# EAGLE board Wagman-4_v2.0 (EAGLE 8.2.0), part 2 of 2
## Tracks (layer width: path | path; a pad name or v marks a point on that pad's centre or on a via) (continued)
INA3  (via drill 0.3 pad 0.61) (continued)
  Bottom 0.254: SWS001.5 6.7,84.12 R103.1
JTAG_RESET
  Top 0.406: RN1.4 29.06,98.05 R41.1 29.14,96.2 JTAG.10
JTAG_TCK  (via drill 0.3 pad 0.61)
  Top 0.2: U1.28 49.49,72.84 v50.25,73.59
  Top 0.254: JTAG.4 25.07,96.5 26.06,97.5 RN1.2
  Bottom 0.2: JTAG.4 25.07,96.5 26.84,98.28 45.84,98.28 49.88,94.24 49.88,75.59 50.49,74.98 50.49,73.83 v50.25,73.59
JTAG_TDI  (via drill 0.3 pad 0.61)
  Top 0.2: U1.29 47.17,73.34
  Top 0.203: 47.17,73.34 46.87,73.34 v46.76,73.45
  Top 0.254: JTAG.8 27.61,96.61 26.86,97.36 RN1.3
  Bottom 0.2: JTAG.8 27.61,97.05 27.94,97.38 45.34,97.38 48.94,93.78 48.94,74.78 47.78,73.61
  Bottom 0.203: 47.78,73.61 47.61,73.45 v46.76,73.45
JTAG_TDO  (via drill 0.3 pad 0.61)
  Top 0.2: U1.30 49.33,73.84 49.71,74.22 v49.76,74.5
  Bottom 0.2: JTAG.6 26.34,96.88 27.24,97.78 45.64,97.78 49.37,94.05 49.37,74.93 v49.76,74.5
JTAG_TMS  (via drill 0.3 pad 0.61)
  Top 0.2: U1.31 47.11,74.34
  Top 0.203: 47.11,74.34 46.24,74.34 v46.11,74.2
  Top 0.254: JTAG.2 23.79,96.58 RN1.1
  Bottom 0.2: 34.3,96.68 45.24,96.68 48.44,93.48 48.44,75.48 47.65,74.69 | 22.14,95.48 22.59,95.93 JTAG.2
  Bottom 0.203: 34.3,96.68 30.84,96.68 30.27,96.11 30.27,94.48 29.15,93.37 22.45,93.37 22.14,93.67 22.14,95.48 | 47.65,74.69 47.17,74.2 v46.11,74.2
LED0  (via drill 0.3 pad 0.61)
  Top 0.2: U1.68 30.86,75.66 v34.59,71.93
  Top 0.254: R14.1 129.71,88.2 124.23,82.72 107.49,82.72 105.79,82.72 v102.43,79.37
  Bottom 0.2: 62.68,74.87 59.33,71.52 45,71.52 43.48,73.05 35.71,73.05 v34.59,71.93
  Bottom 0.203: v102.43,79.37 101.75,78.68 91.64,78.68 90.57,77.62 71.22,77.62 68.47,74.87 62.68,74.87
LED1  (via drill 0.3 pad 0.61)
  Top 0.254: U1.144 46.36,56.56 v46.84,56.08 | R88.1 113.38,85.06 v113.33,85.01
  Bottom 0.254: v113.33,85.01 107.59,79.27 107.59,69.29 100.48,62.17 91.13,62.17 85.52,56.56 47.31,56.56 v46.84,56.08
LED2  (via drill 0.3 pad 0.61)
  Top 0.254: U1.139 43.86,56.46 44.94,55.38 v46.04,55.38 | R15.1 115.54,85.95 v114.47,84.88
  Bottom 0.254: v46.04,55.38 46.34,55.08 47.84,55.08 48.81,56.05 86.01,56.05 91.53,61.57 100.78,61.57 108.3,69.08 108.3,78.71 v114.47,84.88
LED3  (via drill 0.3 pad 0.61)
  Top 0.254: U1.136 42.36,56.36 43.54,55.18 v44.04,55.18 | R89.1 117.57,86.71 v115.62,84.75
  Bottom 0.254: v44.04,55.18 44.84,55.18 45.57,54.45 48.36,54.45 49.45,55.55 86.51,55.55 91.92,60.96 101.09,60.96 109.01,68.88 109.01,78.15 v115.62,84.75
LED4  (via drill 0.3 pad 0.61)
  Top 0.254: U1.135 41.86,55.96 43.64,54.18 v44.44,54.18 | R37.1 119.61,87.22 v117.14,84.75
  Bottom 0.254: v44.44,54.18 44.94,53.68 48.47,53.68 49.7,54.91 86.87,54.91 92.31,60.35 101.39,60.35 109.72,68.68 109.72,77.62 116.86,84.75 v117.14,84.75
LED5  (via drill 0.3 pad 0.61)
  Top 0.254: U1.134 41.36,55.56 v43.54,53.38 | R90.1 121.51,87.73 v118.54,84.75
  Bottom 0.254: v43.54,53.38 43.84,53.08 48.76,53.08 50.08,54.4 87.46,54.4 92.8,59.74 101.7,59.74 110.33,68.37 110.33,77.27 116.93,83.87 117.65,83.87 v118.54,84.75
LED6  (via drill 0.3 pad 0.61)
  Top 0.254: U1.133 40.86,54.96 v42.34,53.48 | R91.1 123.4,87.97 v120.06,84.63
  Bottom 0.254: v42.34,53.48 43.34,52.48 49.18,52.48 50.59,53.89 87.85,53.89 93.09,59.13 102,59.13 110.94,68.07 110.94,76.91 117.14,83.1 118.54,83.1 v120.06,84.63
LED7  (via drill 0.3 pad 0.61)
  Top 0.254: U1.132 40.36,54.26 v42.24,52.38 | R92.1 125.45,88.62 v121.46,84.63
  Bottom 0.254: v42.24,52.38 42.84,51.78 49.49,51.78 51.1,53.39 88.45,53.39 93.58,58.52 102.31,58.52 111.55,67.76 111.55,76.49 117.53,82.47 119.3,82.47 v121.46,84.63
LED8  (via drill 0.3 pad 0.61)
  Top 0.2: U1.20 56.14,68.84 64.94,77.64 67.74,77.64 v67.99,77.39
  Top 0.254: R93.1 111.22,89.63 v102.05,80.46
  Bottom 0.203: v102.05,80.46 100.73,79.14 91.13,79.14 90.22,78.23 70.71,78.23 69.87,77.39 v67.99,77.39
LED9  (via drill 0.3 pad 0.61)
  Top 0.2: U1.21 55.87,69.34 64.69,78.15 v68.75,78.15
  Top 0.254: R94.1 108.94,88.74 v102,81.81
  Bottom 0.2: 101.53,81.34 v102,81.81
  Bottom 0.203: v68.75,78.15 69.44,78.84 89.91,78.84 90.83,79.75 99.94,79.75 101.53,81.34
LOPS  (via drill 0.3 pad 0.61)
  Top 0.254: v105.84,39.54 105.84,30.53 99.87,24.56 92.81,24.56 90.72,22.47 v90.72,21 | v69.29,10.21 69.14,10.05 R97.2 | U17.11 116.59,68.16 v116.58,68.14 | v105.05,43.89 105.46,44.29 v105.46,46.12
  Top 0.406: JP3.2 67.97,9.9 R97.2
  Bottom 0.254: v90.72,21 90.72,12.11 88.82,10.21 v69.29,10.21 | v116.58,68.14 116.56,68.12 114.55,68.12 103.37,56.94 103.37,48.2 v105.46,46.12 | v105.05,43.89 105.84,43.1 v105.84,39.54
MASTER-RESET  (via drill 0.3 pad 0.61)
  Top 0.2: U1.47 41.36,84.03 43.58,86.25 v43.58,87.17 | v45.92,93.87 45.92,87.57 v46.33,87.17
  Top 0.254: J11.5 v7.34,86.5 36.51,86.5 36.98,86.96 36.98,90.11 37.99,91.13 41.35,91.13 v43.99,93.77 43.64,94.12 43.64,98.48 C41.2 43.99,98.55 | v82.68,81.58 82.74,81.58 83.71,80.61 83.71,78.13 83.98,77.86 U24.1 84.73,77.21 v85.44,76.5 | v136.95,84.22 136.44,84.22 v135.22,83 | v106.88,78.23 v105.25,78.23 | v51.3,86.05 50.59,86.76 46.73,86.76 v46.33,87.17
  Top 0.406: C41.2 RST.2 | R41.2 31.67,98.69 RST.1
  Top 0.61: RST.1 RST.2
  Bottom 0.254: v43.58,87.17 v46.33,87.17 | v51.3,86.05 52.32,85.03 69.39,85.03 72.84,81.58 v82.68,81.58 | v45.92,93.87 45.82,93.77 v43.99,93.77 | U39.4 138.37,85.64 v136.95,84.22 | v135.22,83 125.98,83 122.93,86.05 112.77,86.05 106.88,80.16 v106.88,78.23 | v85.44,76.5 93.77,76.5 95.09,77.82 101.8,77.82 102.51,78.53 104.95,78.53 v105.25,78.23
MFP
  Top 0.406: U2.7 98.83,80.29 R20.1
MR1
  Top 0.254: R4.1 98.09,69.33 Q8.3 98.17,68.64 100.35,66.47 SWS003.1
MR1_3V  (via drill 0.3 pad 0.61)
  Top 0.203: U1.32 46.97,74.84 v46.73,75.08
  Top 0.254: v95.09,81.68 96.01,80.77 96.01,74.16 96.31,73.86 v96.31,72.64 | R3.1 98.36,65.29 Q8.2 98.24,66.55 97.23,67.56 96.52,67.56 96.21,67.86 v96.21,68.88 | v52.22,86.56 51.3,87.47 v47.75,87.47
  Bottom 0.203: v47.75,87.47 47.98,87.24 47.98,76.33 v46.73,75.08
  Bottom 0.254: v96.31,72.64 96.31,68.98 v96.21,68.88 | v52.22,86.56 53.13,85.64 69.9,85.64 73.05,82.49 83.19,82.49 84,81.68 v95.09,81.68
MR2
  Top 0.3: Q1.3 103.67,69.38 103.17,68.88 103.17,65.96 102.66,65.45 101.9,65.45 101.57,65.78 SWS003.2
  Top 0.5: R96.1 105.12,70.26 Q1.3
MR2_3V  (via drill 0.3 pad 0.61)
  Top 0.2: U1.22 55.61,69.84 64.94,79.17 69.13,79.17 | 77.24,76.88 80.82,73.3 v81.94,73.3
  Top 0.203: 69.13,79.17 71.29,77.01 77.11,77.01 77.24,76.88
  Top 0.254: R95.1 106.07,65.95 Q1.2 106.09,67.28 106.09,73.07 105.71,73.45 v97.96,73.45
  Bottom 0.2: v97.96,73.45 82.19,73.45 v81.94,73.3
N$1
  Top 0.254: ON.A 134.03,95.02 133.6,94.58 133.6,92.65 133.97,92.29 RN3.4
N$2
  Bottom 0.254: U37.3 83.76,90.77 83.31,91.23 83.31,92.96 83,93.26 R102.2
N$3
  Top 0.406: L.A R15.2
N$4
  Top 0.406: TX1.A R14.2
N$5
  Top 0.2: U1.51 39.36,79.9 39.86,80.4 39.86,83.88 39.22,84.51 R5.1
N$6
  Top 0.406: R33.2 76.52,64.06 76.74,64.28 77.77,64.28 U18.1
N$7
  Top 0.254: R10.2 37.31,80.94 38.36,79.89 U1.53
N$8
  Top 0.406: U6.4 104.45,19.26 R64.2
N$9
  Top 1.93: F1.1 L6.2
N$10
  Top 0.406: ON1.A R2.2
N$11
  Top 0.2: R6.1 50.58,78.12 49.84,77.38 47.66,77.38 46.78,76.5 44.6,76.5 44.19,76.91 44.19,77.62 43.99,77.82 43.58,77.82 43.36,78.04 U1.43
N$12  (via drill 0.3 pad 0.61)
  Top 0.2: R7.1 47.49,80.43 | U1.42 43.86,80.6 v44.35,81.09
  Top 0.203: 47.49,80.43 46.98,80.43 v46.93,80.48
  Bottom 0.2: v46.93,80.48 44.96,80.48 v44.35,81.09
N$13
  Top 0.5: U25.10 67.57,86.02 R28.1
N$14
  Top 0.254: U20.13 83.42,65.64 83.74,65.32 83.74,62.3 R18.1
N$15
  Top 0.406: U2.2 98.83,91.05 Y3.P$4 97.4,92.04 C15.1
N$16
  Top 0.61: JP9.2 27.29,88.64 U36.3
N$17
  Top 0.406: U2.1 100.1,91.1 Y3.P$1 101.5,92.04 C14.1
N$18
  Top 0.254: U26.3 90.64,71.09 R25.1
N$19  (via drill 0.3 pad 0.61)
  Top 0.254: U21.10 71.23,39.39 v71.24,39.38
  Bottom 0.254: R60.2 71.11,39.25 v71.24,39.38
N$20
  Top 0.203: U20.10 84.49,69.45 85.54,70.51 85.54,72.33 84.15,73.73 R19.1
N$21
  Top 0.813: R21.2 104.83,91.06 D3.K
N$22
  Top 0.406: L7.A R88.2
N$23
  Top 0.61: JP9.1 27.29,91.18 U36.4
N$24
  Top 0.406: U20.4 89.93,68.18 R23.2
N$25
  Top 0.406: L4.A R37.2
N$28
  Top 0.254: U18.4 76.69,68.06 76.37,68.37 76.37,73.33 R34.2
N$29  (via drill 0.3 pad 0.61)
  Top 0.2: v53.89,37.64 53.89,38.76 R38.1
  Top 0.254: J5.1 108.99,13.16 111.93,16.1 v111.93,20.49 | v70.66,24.3 70.15,24.81 70.15,30.32 73.76,33.93 v73.76,36.47
  Bottom 0.254: v111.93,20.49 108.12,24.3 v70.66,24.3 | v53.89,37.64 54.64,37.64 55.81,36.47 v73.76,36.47
N$30
  Top 0.2: U18.10 71.48,69.33 71.22,69.59 71.22,73.76 R35.1
N$31  (via drill 0.3 pad 0.61)
  Top 0.2: v103.93,10.08 103.93,7.54 J5.3 | R39.1 57.4,34.37 57.4,27.73 54.71,25.04 54.71,19.64 55.97,18.38 55.97,15.49 v57.07,14.4
  Bottom 0.2: v57.07,14.4 59.48,11.98 62.4,11.98 65.2,9.19 75.74,9.19 76.88,8.05 101.9,8.05 v103.93,10.08
N$32  (via drill 0.3 pad 0.61)
  Top 0.254: J6.1 86.89,13.74 88.18,15.03 88.24,15.08 88.24,19.18 87.64,19.78 87.64,22.74 v92.5,27.61 | v88.31,29 89.2,29.89 89.2,41.78 v90.01,42.59 | R40.1 68.25,47.7 v68.47,47.7
  Bottom 0.254: v92.5,27.61 91.11,29 v88.31,29 | v90.01,42.59 83.48,42.59 82.7,43.38 72.54,43.38 71.01,44.9 71.01,46.83 70.15,47.7 v68.47,47.7
N$33  (via drill 0.3 pad 0.61)
  Top 0.2: J6.3 81.89,13.07 76.25,18.71
  Top 0.254: 76.25,18.71 70.66,18.71 68.37,21 68.37,23.61 69.52,24.75 69.52,30.7 72.2,33.38 72.2,36.13 74.06,37.99 74.06,39.11 v74.47,39.52
  Bottom 0.254: R24.1 74.28,39.33 v74.47,39.52
N$34
  Top 0.254: J7.1 53.26,7.45 53.26,6.52 53.55,6.23 60.83,6.23 61.15,6.55 61.15,8.41 63.81,11.08 R42.1
N$35  (via drill 0.3 pad 0.61)
  Top 0.254: J7.3 48.29,9.94 v48.43,10.08 | R43.1 62.07,10.89 v62.02,10.84
  Bottom 0.254: v48.43,10.08 56.94,10.08 57.58,9.44 60.24,9.44 61.64,10.84 v62.02,10.84
N$36  (via drill 0.3 pad 0.61)
  Top 0.254: R44.1 60.48,10.85 v60.5,10.84 | v31.16,10.59 31.16,7.51 J8.1
  Bottom 0.254: v60.5,10.84 59.74,10.08 58.34,10.08 56.18,12.24 32.81,12.24 v31.16,10.59
N$37  (via drill 0.3 pad 0.61)
  Top 0.254: R45.1 v58.85,10.84 | v26.21,10.46 26.21,7.5 J8.3
  Bottom 0.254: v58.85,10.84 56.43,13.25 29,13.25 v26.21,10.46
N$38  (via drill 0.3 pad 0.61)
  Top 0.2: R46.1 53.67,52.14 51.99,50.47 51.99,45 52.88,44.12 52.88,31.41 v55.42,28.88
  Top 0.254: J9.1 131.09,13.36 131.87,14.14 134.16,14.14 135.81,15.79 v135.81,24.05
  Bottom 0.254: v135.81,24.05 133.65,26.21 71.93,26.21 68.88,29.26 55.8,29.26 v55.42,28.88
N$39  (via drill 0.3 pad 0.61)
  Top 0.2: v51.99,43.73 51.48,44.24 51.48,57.18 R47.1
  Top 0.254: J9.3 126.09,10.65 v126.03,10.71 | v60.75,28.49 60.75,36.49 61.82,37.56 v61.82,37.9
  Bottom 0.254: v126.03,10.71 126.03,22.65 123.11,25.57 71.67,25.57 68.75,28.49 v60.75,28.49 | v51.99,43.73 54.94,40.78 60.34,40.78 61.82,39.3 v61.82,37.9
N$40
  Top 0.61: U36.1 16.89,91.18 arc90 R31.1
N$42  (via drill 0.3 pad 0.61)
  Top 0.406: J4.2 9.23,38.59 9.04,38.4 v8.94,38.4
  Bottom 0.406: U14.4 U13.3 v8.94,38.4
N$43  (via drill 0.3 pad 0.61)
  Top 0.406: J4.1 9.19,41.09 v9.04,40.94
  Bottom 0.406: U13.4 9.03,40.95 v9.04,40.94
N$44  (via drill 0.3 pad 0.61)
  Top 0.406: J4.3 12.62,34.97 11.68,34.03 v10.16,34.03
  Bottom 0.406: U14.3 10.11,33.99 arc90 v10.16,34.03
N$45
  Top 0.254: R36.1 71.06,62.46 71.06,65.18 71.4,65.52 U18.13
N$46  (via drill 0.3 pad 0.61)
  Top 0.305: U19.1 69.77,63.9 v69.77,61.92
  Top 0.406: R48.2 64.49,62.63 v64.87,63.04
  Bottom 0.305: v64.87,63.04 65.17,63.04 66.29,61.92 v69.77,61.92
N$47
  Top 0.2: U19.4 69.96,68.06 70.66,68.75 70.66,72.31 70.15,72.82 68.95,72.82 R49.2
N$48
  Top 0.406: U19.10 61.95,69.33 R50.1
N$49
  Top 0.254: U19.13 62.08,65.52 R52.1
N$50
  Top 0.254: U25.3 58.01,88.56 R54.2
N$51
  Top 0.254: U25.2 57.7,89.83 C43.1
N$52
  Top 0.254: U25.1 58.47,91.1 R53.2
N$53
  Top 0.5: R53.1 C43.2 R54.1
N$54
  Top 0.406: RN3.1 137.26,94.34 138.09,95.17 RX.A
N$55
  Top 0.406: RN3.2 136.46,94.01 136.19,94.28 TX.A
N$56  (via drill 0.3 pad 0.61)
  Top 0.254: U22.10 61.14,38.39 v60.67,37.92
  Top 0.305: 61.16,39.42 U22.10
  Bottom 0.254: R59.2 59.22,39.37 v60.67,37.92
N$57
  Top 0.406: U16.4 123.46,77.15 R11.2
N$58
  Top 0.406: U23.1 U24.3
N$59
  Top 0.406: R61.1 U23.4
N$60
  Top 0.254: U24.4 80.36,79.76 R62.1
N$63
  Top 0.254: IC1.10 72.29,89.83 75.03,92.58 79.14,92.58 83.68,97.12 91.13,97.12 93.62,99.61 126.67,99.61 127.55,98.72 ACT.A
N$64
  Top 0.254: IC1.2 80.74,83.48 88.79,91.53 X7.5
N$65  (via drill 0.3 pad 0.61)
  Top 0.254: R79.1 127.55,87.99 122.92,83.36 106.45,83.36 v106.3,83.52 | X7.2 85.49,92.09 81.44,88.04 v81.44,88.01 80.88,88.56 IC1.6
  Bottom 0.254: v81.44,88.01 82.98,88.01 86.05,84.93 90.01,84.93 91.43,83.52 v106.3,83.52
N$66
  Top 0.406: ACT.C R79.2
N$67
  Top 0.254: IC1.4 80.82,86.02 86.59,91.8 X7.3
N$68
  Top 0.406: L8.A R89.2
N$69
  Top 0.406: L9.A R90.2
N$70
  Top 0.406: L10.A 123.4,96.48 R91.2
N$71
  Top 0.406: L11.A R92.2
N$72
  Top 0.406: L12.A R93.2
N$73
  Top 0.406: L13.A R94.2
N$74
  Bottom 0.254: U37.2 84.02,89.5 82.8,90.72 82.73,90.72 C1.1
N$75
  Bottom 0.254: U37.1 84.07,88.23 82.9,89.4 R101.2
N$76
  Bottom 0.406: R101.1 80.22,89.71 C1.2 R102.1
N$77
  Top 0.406: U3.4 R13.2
N$78
  Top 0.406: U7.4 R9.2
N$79
  Top 0.406: U8.4 R29.2
N$80
  Top 0.406: U9.4 R30.2
N$81
  Bottom 0.254: U37.10 92.26,93.31 R105.1
N$82
  Bottom 0.406: U38.2 141.75,88.21 R106.1
N$83
  Bottom 0.406: U39.2 135.43,88.18 136.01,88.77 R107.1
N$84
  Bottom 0.254: U40.3 95.48,89.96 R109.2
N$85
  Bottom 0.254: C3.1 U40.2
N$86
  Bottom 0.254: U40.1 95.38,87.42 R108.2
N$87
  Bottom 0.254: R109.1 C3.2 R108.1
N$88
  Bottom 0.406: U40.10 101.54,92.5 100.92,91.88 R112.1
N$89
  Bottom 0.406: U41.4 145.74,78.77 R113.2
NC_AUTO
  Top 0.2: U20.5 85.2,69.45 84.63,68.88 84.63,63.29 90.33,57.59 U10.1
NC_AUTO_DISABLE  (via drill 0.3 pad 0.61)
  Top 0.2: v34.97,65.45 37.07,63.36 v37.07,63.25 | U1.97 28.51,64.84 v29.13,65.45
  Top 0.406: U20.1 87.83,63.93 v87.14,63.24
  Bottom 0.2: v34.97,65.45 v29.13,65.45 | v37.07,63.25 37.07,63.89 39.01,65.83 63.5,65.83 66.31,63.02 83.34,63.02 84.83,64.51 84.83,64.55 R22.2
  Bottom 0.406: R22.2 85.41,64.04 86.2,63.24 v87.14,63.24
NC_BOOT_SEL  (via drill 0.3 pad 0.61)
  Top 0.254: v17.54,84.38 17.74,84.58 29.1,84.58 30.48,83.21 30.48,80.67 31.36,79.78 U1.67 | v16.84,88.49 R31.2
  Bottom 0.254: v17.54,84.38 16.84,85.08 v16.84,88.49
NC_ERASE_MR1  (via drill 0.3 pad 0.61)
  Top 0.254: Q4.3 10.94,67.71 5.18,67.71 4.47,68.42 4.47,78.23 4.77,78.53 7.21,78.53 8.12,79.45 8.12,80.67 v8.02,80.87
  Top 0.305: R118.1 12.46,68.05 Q4.3
  Bottom 0.254: SWS001.1 7.2,81.69 v8.02,80.87
NC_ERASE_MR1_3V
  Top 0.305: R117.1 12.22,64.66 Q4.2
  Top 0.406: R117.1 12.17,63.48 11.88,63.19 7.82,63.19 6.14,64.87 J2.1
NC_ERASE_MR2  (via drill 0.3 pad 0.61)
  Top 0.254: R120.1 9.95,79.24 v9.14,80.06
  Top 0.305: Q5.3 11.58,78.85 R120.1
  Bottom 0.254: SWS001.2 6.7,81.07 7.62,80.16 9.04,80.16 v9.14,80.06
NC_ERASE_MR2_3V
  Top 0.305: Q5.2 12.53,74.01 R119.1 12.38,72.93 11.58,72.13 11.58,70.71 9.85,68.98 J2.2
NC_FET_ATMEL  (via drill 0.3 pad 0.61)
  Top 0.203: U20.8 82.94,71.99 83.31,71.62 v84.83,71.62
  Bottom 0.203: v84.83,71.62 85.03,71.83 88.08,71.83 88.49,71.42 88.49,70.3 88.18,70 J1.2
NC_FET_AUTO  (via drill 0.3 pad 0.61)
  Top 0.203: U20.6 86.67,70.72 v86.15,70.2
  Bottom 0.203: J1.1 86.59,69.05 86.15,69.49 v86.15,70.2
NC_FET_CTRL  (via drill 0.3 pad 0.61)
  Top 0.254: R30.1 123.71,18.02 122.42,19.3 115.41,19.3 114.35,20.37 114.35,39.67 115.11,40.43 115.11,43.07 112.77,45.41 112.77,52.12 111.76,53.13 106.57,53.13 106.19,53.51 98.27,53.51 97.73,54.05 v97.73,54.15 | v94.38,66.54 94.38,57.6 v95.5,56.48
  Bottom 0.254: J1.4 R121.1 92.32,70.94 94.38,68.88 v94.38,66.54 | v95.5,56.48 95.5,56.38 v97.73,54.15
NC_LAT_CLK  (via drill 0.3 pad 0.61)
  Top 0.2: U1.55 37.36,76.63 42.26,71.73 v42.26,71.29 | U20.11 82.44,68.19 v83.74,68.19
  Bottom 0.2: v42.26,71.29 43.25,70.3 60.78,70.3 62.4,71.93 73.66,71.93 | R55.2 84.37,68.19 v83.74,68.19
  Bottom 0.203: 73.66,71.93 82.09,71.93 83.74,70.28 v83.74,68.19
NC_LAT_D  (via drill 0.3 pad 0.61)
  Top 0.2: U20.12 v83.74,66.92 | U1.59 35.36,76.88 40.97,71.27 v41.19,71.27
  Bottom 0.2: v41.19,71.27 42.56,69.9 61.26,69.9 62.78,71.42 73.25,71.42
  Bottom 0.203: v83.74,66.92 83.54,66.92 82.8,67.66 82.8,70.51 81.89,71.42 73.25,71.42
NC_PCMR_MR1
  Bottom 0.254: Q2.3 R114.1 13.19,73.54 13.81,74.16 13.81,80.77 12.85,81.73 SWS002.1
NC_PCMR_MR1_3V
  Bottom 0.254: J2.3 6.23,71.44 Q2.2 9.56,71.39 R26.1
NC_PCMR_MR2
  Bottom 0.254: SWS002.2 10.66,80.97 9.95,80.26 Q3.3 9.93,79.14 R116.1
NC_PCMR_MR2_3V
  Bottom 0.254: J2.4 7.92,74.06 8.83,74.98 R115.1 9.05,76.97 Q3.2
NC_RELAY_CTRL
  Top 0.2: 81.06,69.18 81.06,59.88 81.58,59.36 87.68,59.36 89.06,57.97 U10.2
  Top 0.203: U20.9 81.98,70.72 81.06,69.8 81.06,69.18
NC_RELAY_RETURN  (via drill 0.3 pad 0.61)
  Top 0.254: K1.1 114.6,16.3 113.71,17.19 113.71,42.46 v113.97,42.72 | v91.36,45.64 U10.18 U10.17
  Bottom 0.254: v91.36,45.64 92.25,46.53 103.83,46.53 107.64,42.72 v113.97,42.72
OP1
  Top 0.406: U9.5 U9.6 | U9.8 U9.7
  Top 1.27: 131.29,16.38 K1.S | U9.6 U9.7
  Top 1.5: J9.2 128.59,15.73 129.24,16.38 131.29,16.38 | K1.S 131.36,19.07 U9.6
OP1_ADC  (via drill 0.3 pad 0.61)
  Top 0.2: U1.79 29.38,73.84 38.27,64.94 v39.89,64.94
  Top 0.254: R67.1 116.87,37.25 116.24,37.88 116.24,43.18 113.74,45.68 113.74,52.68 112.4,54.02 99.11,54.02 98.06,55.06 97.23,55.06 93.77,51.61 69.13,51.61 62.66,58.09 v62.66,59.79
  Top 0.61: R67.1 R68.2
  Bottom 0.2: v62.66,59.79 62.68,59.81 62.68,60.24 61.77,61.16 56.48,61.16 53.33,64.31 46.53,64.31 45.51,65.32 40.27,65.32 v39.89,64.94
OP1_SRC
  Top 0.406: U29.1 115.19,50.76 115.23,50.72 115.62,50.72 115.74,50.85 115.83,50.76 U29.2 | 119.6,40.88 121.25,40.88 121.38,41.02
  Top 0.61: R67.2 119.6,40.88 124.44,40.88
  Top 1.676: X2.3 121.52,40.88 121.38,41.02 115.74,46.66 115.74,50.85
OP2
  Top 0.406: U6.8 107.52,21.2 107.54,21.18
  Top 0.61: 107.54,21.18 107.54,20.62 U6.7 U6.6 U6.5
  Top 1.5: J5.2 106.49,13.13 108.38,15.02 K2.S
  Top 1.676: K2.S 108.38,19.07 U6.6
OP2_ADC  (via drill 0.3 pad 0.61)
  Top 0.2: U1.81 29.62,72.84 38.4,64.05 v39.28,64.05
  Top 0.254: v61.62,60.03 61.62,57.86 68.5,50.97 93.95,50.97 95.98,53.01 105.2,53.01 105.96,52.24 105.96,47.9 101.95,43.89 v101.9,43.89
  Bottom 0.2: v39.28,64.05 40.94,64.05 43.94,61.06 52.52,61.06 53.23,60.35 61.3,60.35 v61.62,60.03
  Bottom 0.254: v101.9,43.89 100.87,42.85 R69.1 100.86,41.91 R73.2
OP2_SRC
  Top 0.406: U30.1 107.71,50.58 108.14,50.83 108.62,50.58 U30.2
  Top 1.676: 108.14,50.83 108.14,44.5 104.52,40.88 X3.3
  Bottom 0.508: R69.2 102.99,40.02 X3.3
OP3
  Top 0.406: U7.8 U7.7 U7.6 | U7.6 U7.5 83.87,19.81 83.87,19.86 83.94,19.93 U7.6
  Top 1.5: J6.2 84.39,13.93 85.39,14.93 K3.S
  Top 1.676: K3.S 85.39,19.61 U7.7
OP3_ADC  (via drill 0.3 pad 0.61)
  Top 0.2: U1.83 29.73,71.84 v38.3,63.27
  Top 0.254: v69.64,46.68 69.64,48 60.75,56.89 v60.75,59.48
  Bottom 0.2: v60.75,59.48 52.47,59.48 51.41,60.55 43.45,60.55 40.74,63.27 v38.3,63.27
  Bottom 0.254: v69.64,46.68 69.64,44.95 72.54,42.06 76.19,42.06 R74.2 78.17,42.01 R70.1
OP3_SRC  (via drill 0.71 pad 1.63)
  Top 0.406: U32.2 100.5,50.76 U32.1
  Top 1.676: 100.5,50.76 100.5,50.34 v92.73,42.57
  Bottom 0.406: R70.2 80.11,40.12 X4.3
  Bottom 1.676: X4.3 90.97,40.88 92.65,42.57 v92.73,42.57
OP4
  Top 0.5: U3.6 U3.5
  Top 1.5: K4.S 51.74,16.3 | 51.74,16.3 50.02,16.3 47.16,19.16 | 47.16,19.16 U3.6 U3.7 U3.8 | 47.16,19.16 47.14,19.18 47.14,20.18 | J7.2 50.79,15.35 51.74,16.3
OP4_ADC
  Top 0.2: U1.85 29.2,70.84 31.54,68.5 31.54,61.98 27.74,58.18 27.74,56.08 28.35,55.47 30.58,55.47 30.98,55.06 30.98,52.42 32.71,50.69 38.63,50.69 39.67,51.73 40.51,51.73 41.35,50.9 43.78,50.9 44.62,50.06 44.62,44.62 41.58,41.58 38.63,41.58
  Top 0.203: 38.63,41.58 37.61,41.58 36.98,40.94 36.98,38.71 37.46,38.23 R71.1
  Top 1: R71.1 R75.2
OP4_SRC
  Top 0.406: U33.1 47.25,44.46 47.29,44.5 47.85,44.5 U33.2
  Top 1: R71.2 43.17,40.13
  Top 1.016: 43.17,40.13 46.96,40.13 X5.3
  Top 1.676: X5.3 47.29,41.77 47.29,44.5
OP5
  Top 0.61: 28.07,19.55 U8.5
  Top 1.27: 28.07,19.55 U8.6 U8.7 U8.8
  Top 1.5: J8.2 28.69,13.73 29.24,14.28 K5.S 29.24,18.38 28.07,19.55
OP5_ADC  (via drill 0.3 pad 0.61)
  Top 0.2: U1.89 21.4,68.84 19.64,67.08 19.64,62.44 18.71,61.51 18.71,53.06 17.88,52.22 17.88,51.2 18.08,51 18.59,51 22.35,47.24 22.35,46.43
  Top 0.203: 22.35,46.43 22.35,43.58 22.75,43.18 v24.68,43.18
  Bottom 0.203: v24.68,43.18 26.93,43.18 R72.1
  Bottom 0.406: R72.1 R76.2
OP5_SRC
  Top 0.61: U34.2 26.92,44.46 U34.1
  Top 1.676: X6.3 26.92,43.08 26.92,44.46
  Bottom 0.406: R72.2 25.53,40.07 X6.3
OUTY1  (via drill 0.3 pad 0.61)
  Top 0.203: U12.7 32.25,89.12 R66.2
  Top 0.254: U25.6 55.34,84.75 51.91,88.18 v46.93,88.18 | R66.2 32.47,88.08 v31.8,88.08 | v31.8,88.08 31.69,88.08 v31.8,88.08
  Bottom 0.254: v46.93,88.18 46.83,88.08 v31.8,88.08
OUTY2  (via drill 0.3 pad 0.61)
  Top 0.203: v90.32,97.84 88.39,99.77 72.64,99.77 68.68,95.8 v64.51,95.8 | R86.2 29.63,89.81 v25.29,89.81
  Top 0.254: U12.5 30.33,90.03 R86.2
  Bottom 0.203: U40.6 96.01,93.77 91.94,97.84 v90.32,97.84
  Bottom 0.254: v64.51,95.8 49,95.8 46.04,98.76 24.74,98.76 21.13,95.15 21.13,93.47 24.79,89.81 v25.29,89.81
OUTY3  (via drill 0.3 pad 0.61)
  Top 0.203: R65.2 34.91,92.45 v36.57,92.45
  Top 0.254: U12.2 32.25,91.9 32.51,91.64 34.1,91.64 R65.2
  Top 0.305: v50.8,92.86 47.54,92.86 v46.83,92.15
  Bottom 0.2: 46.53,92.45 46.37,92.6 36.72,92.6 v36.57,92.45
  Bottom 0.203: v46.83,92.15 46.53,92.45
  Bottom 0.305: U37.6 79.34,94.58 76.5,91.74 67.25,91.74 65.63,93.37 51.3,93.37 v50.8,92.86
P1RX
  Top 0.2: U1.3 51.22,60.34 R47.2
P1THM  (via drill 0.3 pad 0.61)
  Top 0.2: R85.1 24.56,74.29 24.56,74.34 | v17.45,61.01 v17.45,55.04
  Top 0.254: J9.5 121.09,10.57 v121.08,10.59 | U1.78 24.55,74.34 24.18,73.96 24.18,73.78 R85.1 | 24.56,74.34 24.81,74.34 24.94,74.21 v24.94,73.71
  Bottom 0.2: v17.45,61.01 17.45,61.51 26.46,70.53 26.46,72.82 25.57,73.71 v24.94,73.71
  Bottom 0.254: v121.08,10.59 122.47,11.98 122.47,23.79 121.33,24.94 71.42,24.94 68.5,27.86 61.53,27.86 61.31,27.64 55.33,27.64 54.02,26.33 14.9,26.33 14.12,27.12 14.12,29.15 17.67,32.71 17.67,38.71 22.78,43.81 22.78,50.67 19.6,53.84 18.64,53.84 v17.45,55.04
P1TX
  Top 0.2: U1.4 52.29,60.84 R46.2
P2RX_A
  Top 0.2: U1.5 54.07,61.34 54.78,60.62 54.78,52.37 52.5,50.08 52.5,45.39 54.78,43.1 56.81,43.1 57.24,43.52 U22.17
P2RX_B
  Top 0.254: U22.4 57.24,36.39 R39.2
P2THM  (via drill 0.3 pad 0.61)
  Top 0.2: U1.80 25.84,73.34 v25.07,72.56 25.07,72.31 24.56,71.8 R81.1 | v16.56,60.24 v16.56,54.3
  Top 0.254: J5.5 98.99,12.86 97.45,14.4 v89.33,14.4 | v70.02,15.16 70.02,17.95 v69.9,18.08
  Bottom 0.2: v25.07,72.56 25.95,71.67 25.95,70.78 16.56,61.39 v16.56,60.24
  Bottom 0.254: v89.33,14.4 70.78,14.4 v70.02,15.16 | v69.9,18.08 69.9,20.24 68.63,21.51 68.63,22.91 69.64,23.92 69.64,25.83 68.37,27.1 55.55,27.1 54.02,25.57 14.14,25.57 13.41,26.31 13.41,29.36 17.17,33.12 17.17,38.91 22.02,43.77 22.02,50.41 19.2,53.23 17.62,53.23 v16.56,54.3
P2TX_A
  Top 0.2: U1.6 54.46,61.84 55.29,61.01 55.29,51.99 53,49.7 53,45.64 55.04,43.61 56.31,43.61 56.59,43.89 U22.18
P2TX_B
  Top 0.2: U22.3 56.59,40.66 56.31,40.94 54.47,40.94 R38.2
P3RX_A  (via drill 0.3 pad 0.61)
  Top 0.2: U1.16 56.7,66.84 57.32,66.21 57.32,48.81 v58.21,47.93 | U21.4 66.76,37.93 v66.72,37.89
  Bottom 0.2: v58.21,47.93 58.47,47.67 58.47,46.91 66.72,38.65 v66.72,37.89
P3RX_B  (via drill 0.3 pad 0.61)
  Top 0.254: U21.17 66.76,46.87 v66.47,47.16
  Bottom 0.254: R24.2 72.56,41.07 v66.47,47.16
P3THM  (via drill 0.3 pad 0.61)
  Top 0.2: U1.82 25.85,72.34 25.07,71.55 v25.07,71.04
  Top 0.254: J6.5 76.89,11.47 74.09,14.27 67.93,14.27 | 67.93,14.27 R82.1 | 67.93,14.27 67.93,15.99 v69.01,17.06 | v15.67,53.56 15.67,61.64 v15.79,61.77
  Bottom 0.2: v25.07,71.04 v15.79,61.77
  Bottom 0.254: v69.01,17.06 69.01,20.11 67.86,21.25 67.86,22.91 68.88,23.92 68.88,25.83 68.12,26.59 55.98,26.59 54.2,24.81 13.69,24.81 12.7,25.8 12.7,29.66 16.45,33.42 16.45,39.21 21.38,44.14 21.38,50.14 18.89,52.62 16.61,52.62 v15.67,53.56
P3TX_A  (via drill 0.3 pad 0.61)
  Top 0.2: U1.15 56.31,66.34 56.81,65.83 56.81,48.05 v57.07,47.8 | U21.3 66.11,38.3 65.83,38.02 v65.83,37.26
  Bottom 0.2: v57.07,47.8 57.96,46.91 57.96,46.66 65.26,39.35 65.83,38.78 v65.83,37.26
P3TX_B
  Top 0.254: U21.18 66.11,46.12 65.53,46.71 65.53,48.66 R40.2
P4_FET_CTRL  (via drill 0.3 pad 0.61)
  Top 0.2: U19.6 67.8,70.6 66.98,69.77 66.98,62.55 70.78,58.75 v70.78,57.55
  Top 0.254: R13.1 35.94,18.92 34.84,20.01 34.84,39.11 v35.66,39.92
  Bottom 0.2: 37.38,41.96 39.67,44.24 39.67,52.12 44.62,57.07 70.3,57.07 v70.78,57.55
  Bottom 0.203: 37.38,41.96 35.66,40.23 v35.66,39.92
P4_LAT_CLK  (via drill 0.3 pad 0.61)
  Top 0.2: U19.3 v68.27,66.79 v68.26,66.78 | U1.65 32.36,76.19 37.69,70.86 37.69,69.76 v38.46,68.99
  Bottom 0.2: v68.26,66.78 68.26,68.61 67.48,69.39 64.31,69.39 63.19,68.27 39.18,68.27 v38.46,68.99
  Bottom 0.203: R99.1 78.33,66.14 77.31,67.15 75.18,67.15 74.06,66.03 69,66.03 v68.26,66.78
P4_LAT_D  (via drill 0.3 pad 0.61)
  Top 0.2: v68.18,65.53 68.32,65.52 U19.2 | U1.66 31.86,75.93 37.08,70.71 37.08,69.27 v37.39,68.97
  Bottom 0.2: v68.18,65.53 68.04,65.53 67.36,66.21 67.36,68.37 66.85,68.88 64.69,68.88 63.57,67.76 38.59,67.76 v37.39,68.97
P4_RELAY_CTRL
  Top 0.2: U10.5 85.25,56.58 84.88,56.94 79.7,56.94 | U19.5 68.44,69.33 67.46,68.35 67.46,63 70.72,59.74 | 74.67,57.4 73.66,58.41
  Top 0.203: 74.67,57.4 75.13,56.94 79.7,56.94 | 73.66,58.41 72.33,59.74 70.72,59.74
P4_RELAY_RETURN  (via drill 0.3 pad 0.61)
  Top 0.254: K4.1 36.5,16.3 34.23,18.56 34.23,39.92 36.52,42.21 41.32,42.21 43.76,44.65 v43.76,49.07 | U10.14 85.25,46.9 v83.98,48.17
  Bottom 0.254: v43.76,49.07 44.01,49.32 50.85,49.32 52.67,51.15 80.99,51.15 v83.98,48.17
P4RX  (via drill 0.3 pad 0.61)
  Top 0.254: v63.11,14.54 R43.2
  Bottom 0.254: SJ8.1 61.88,24.03 61.64,23.79 61.64,22.52 | SJ8.3 61.76,22.4 61.64,22.52 | 64.31,17.57 64.31,15.92 64.12,15.73 SJ6.1 63.11,14.67 v63.11,14.54 | 64.31,17.57 64.31,18.71 63.98,19.05 SJ7.3 62.07,19.05 61.64,19.48 61.64,20.87 | 61.64,20.87 61.64,22.52 | SJ7.1 61.84,20.67 61.64,20.87 | SJ6.3 64.09,17.36 64.31,17.57
P4RX_A  (via drill 0.3 pad 0.61)
  Top 0.2: U1.18 57.35,67.84 58.31,66.87 58.31,50.19 59.48,49.02 59.48,47.04 58.54,46.09 U22.15 58.54,42.14 58.97,41.7 66.98,41.7 68.06,40.62 U21.6
  Top 0.254: U21.6 68.06,36.06 63.55,31.54 63.55,23.16 | 63.55,23.16 63.55,22.65 | v64.41,21.55 63.55,22.41 63.55,23.16
  Bottom 0.254: SJ7.2 64.06,19.86 64.41,20.21 v64.41,21.55
P4RX_B_1.8  (via drill 0.3 pad 0.61)
  Top 0.254: U22.6 58.54,26.13 55.67,23.26 55.67,19.4 56.9,18.17 v61.79,18.17
  Bottom 0.254: SJ6.2 62.04,16.54 61.79,16.79 v61.79,18.17
P4RX_B_5  (via drill 0.3 pad 0.61)
  Top 0.254: U21.15 68.06,43.79 70.1,41.75 71.33,41.75 72.54,40.54 72.54,38.7 70.67,36.83 70.67,34.48 67.61,31.41 67.61,25.45 v67.36,25.19
  Bottom 0.254: v67.36,25.19 66.98,24.81 65.83,24.81 64.24,23.22 SJ8.2
P4THM  (via drill 0.3 pad 0.61)
  Top 0.2: 37.64,51.61 v37.89,51.86 37.23,51.2 32.81,51.2 31.49,52.52 31.49,55.57 31.09,55.98 28.54,55.98 28.24,56.28 28.24,58.08 32.05,61.89 32.05,68.75 29.47,71.34 U1.84
  Top 0.254: J7.5 43.29,13.19 42.08,14.4 35.48,14.4 32.05,17.83 32.05,26.66 32.91,27.53 32.91,40.91 38.93,46.93 R83.1 38.29,48.69 v37.77,48.69
  Bottom 0.2: v37.89,51.86 37.77,51.73 v37.77,48.69
P4TX  (via drill 0.3 pad 0.61)
  Top 0.254: R42.2 63.81,14.16 v64.18,14.52
  Bottom 0.254: SJ4.3 65.8,24.02 65.58,23.79 65.58,22.65 65.84,22.39 SJ4.1 66.78,20.68 SJ5.1 67.56,20.67 67.99,20.24 67.99,19.22 | 67.99,17.57 67.99,16.18 67.57,15.76 SJ2.3 65.41,15.76 v64.18,14.52 | 67.99,17.57 67.99,19.22 | SJ2.1 67.8,17.38 67.99,17.57 | SJ5.3 67.81,19.04 67.99,19.22
P4TX_A  (via drill 0.3 pad 0.61)
  Top 0.2: U1.17 57.09,67.34 57.81,66.62 57.81,49.83 58.97,48.66 58.97,47.29 57.89,46.2 U22.16 57.89,41.65 58.34,41.19 66.59,41.19 67.41,40.38 U21.5
  Top 0.254: U21.5 67.41,36.37 62.78,31.74 62.78,24.38 59.13,20.72 59.13,19.5 59.66,18.97 64.94,18.97 v65.83,19.87
  Bottom 0.254: v65.83,19.87 65.83,19.86 SJ5.2
P4TX_B_1.8  (via drill 0.3 pad 0.61)
  Top 0.254: U22.5 57.89,27.03 v56.56,25.7
  Bottom 0.254: SJ4.2 67.4,23.2 67.86,23.67 67.86,24.43 68.25,24.81 68.25,25.57 67.74,26.08 56.94,26.08 v56.56,25.7
P4TX_B_5  (via drill 0.3 pad 0.61)
  Top 0.254: U21.16 67.41,43.55 69.72,41.25 71.12,41.25 72.03,40.33 72.03,38.91 70.07,36.95 70.07,34.77 67.33,32.02 66.98,31.67 66.24,30.93 66.24,22.75 66.64,22.35 66.64,19.27 66.47,19.1 v65.49,18.22
  Bottom 0.254: SJ2.2 65.69,16.57 65.49,16.77 v65.49,18.22
P5_FET_CTRL  (via drill 0.3 pad 0.61)
  Top 0.2: U19.8 65.51,71.87 66.47,70.91 66.47,61.9 69.49,58.87 v69.49,58.16 | R29.1 21.92,17.92 20.62,19.22 13,19.22 11.73,20.49 11.73,30.91
  Top 0.203: 11.73,30.91 16.86,36.04 16.86,39.11 19.3,41.55 v21.84,41.55
  Bottom 0.2: 38.91,47.44 38.91,52.12 44.37,57.58 68.91,57.58 v69.49,58.16
  Bottom 0.203: v21.84,41.55 24.48,44.19 31.29,44.19 32.41,43.07 37.59,43.07 38.91,44.39 38.91,47.44
P5_LAT_CLK  (via drill 0.3 pad 0.61)
  Top 0.2: U19.11 65.14,68.06 v65.16,68.08 | U1.100 29.47,63.34 v29.76,63.04
  Bottom 0.2: v29.76,63.04 29.76,64.18 30.14,64.56 35.22,64.56 37.92,67.25 64.33,67.25 v65.16,68.08 66.24,67 66.24,65.53 67.57,64.19 74.36,64.19 76.02,65.86 76.89,65.86 78.03,64.71
  Bottom 0.203: 78.03,64.71 78.54,64.21 R100.1
P5_LAT_D  (via drill 0.3 pad 0.61)
  Top 0.2: U19.12 v65.12,66.79 v65.13,66.78 | U1.99 30.62,63.84 v30.65,63.8
  Bottom 0.2: v30.65,63.8 35.35,63.8 38.33,66.78 v65.13,66.78
P5_RELAY_CTRL
  Top 0.2: U10.6 83.98,56.07 83.61,56.43 79.4,56.43 | U19.9 65,70.6 65.96,69.64 65.96,60.42 69.69,56.69 71.32,56.69 71.62,56.99 | 73.15,58.11 74.27,56.99
  Top 0.203: 74.27,56.99 74.82,56.43 79.4,56.43 | 71.62,56.99 71.62,57.91 71.83,58.11 73.15,58.11
P5_RELAY_RETURN  (via drill 0.3 pad 0.61)
  Top 0.254: v42.95,49.97 42.95,44.73 41.07,42.85 36.04,42.85 33.73,40.53 33.73,27.12 33.33,26.72 v33.33,19.71 | v83.98,43.89 U10.13
  Bottom 0.254: K5.1 22.22,16.3 25.64,19.71 v33.33,19.71 | v83.98,43.89 84.88,44.8 84.88,48.43 81.58,51.73 52.24,51.73 50.48,49.97 v42.95,49.97
P5RX  (via drill 0.3 pad 0.61)
  Top 0.254: R45.2 58.34,13.88 v58.34,14.32
  Bottom 0.254: SJ12.1 54.74,24.09 54.43,23.77 54.43,22.63 | 54.43,22.63 54.43,20.98 | 54.43,20.98 54.43,19.32 | 54.43,19.32 54.43,17.55 54.62,17.35 54.69,17.35 | 54.69,17.35 SJ14.1 | SJ13.1 54.62,19.13 54.43,19.32 | SJ13.3 54.64,20.76 54.43,20.98 | SJ12.3 54.59,22.46 54.43,22.63 | 54.69,17.35 54.69,16.01 54.98,15.73 SJ14.3 57.31,15.73 58.34,14.7 v58.34,14.32
P5RX_A  (via drill 0.3 pad 0.61)
  Top 0.2: U1.14 55.8,65.84 56.31,65.32 56.31,47.42 v57.07,46.66 | U22.13 59.84,43.63 v60.37,43.1 66.98,43.1 69.36,40.71 U21.8
  Top 0.254: U21.8 69.36,35.2 65.07,30.91 v65.07,25.19 | v62,25.22 61.92,25.22 v56.66,19.96
  Bottom 0.2: v57.07,46.66 60.37,43.35 v60.37,43.1
  Bottom 0.203: SJ13.2 v56.66,19.96
  Bottom 0.254: v62,25.22 62.02,25.19 v65.07,25.19
P5RX_B_1.8  (via drill 0.3 pad 0.61)
  Top 0.254: U22.8 59.84,24.79 58.31,23.26 v56.66,23.26
  Bottom 0.254: v56.66,23.26 SJ12.2
P5RX_B_5  (via drill 0.3 pad 0.61)
  Top 0.254: U21.13 69.36,44.01 70.61,42.77 71.75,42.77 73.55,40.96 73.55,38.28 71.69,36.41 71.69,33.59 68.88,30.78 68.88,24.9 67.86,23.89 67.86,18.08 65.58,15.79 57.42,15.79 v56.69,16.53
  Bottom 0.254: v56.69,16.53 SJ14.2
P5THM
  Top 0.2: U1.88 21.2,69.34 19.14,67.28 19.14,62.7 18.21,61.77 18.21,53.25 13.24,48.28 13.24,45.58 | J8.5 21.19,12.94 19.86,14.27 15.54,14.27 9.77,20.04 9.77,30.62 R84.1 9.84,30.76
  Top 0.203: 13.24,45.58 13.24,45.37 16.15,42.46 16.15,36.06 10.81,30.72 R84.1
P5TX  (via drill 0.3 pad 0.61)
  Top 0.254: 60.48,13.69 R44.2 59.33,14.55 v59.33,14.65
  Bottom 0.254: SJ9.1 60.42,24.05 60.57,23.9 60.57,22.63 | 60.57,22.63 60.57,21.23 60.13,20.78 SJ10.3 58.35,20.78 58.16,20.59 58.16,19.32 | SJ9.3 60.37,22.42 60.57,22.63 | 58.16,19.32 58.16,17.67 | 58.16,17.67 58.16,16.15 58.42,15.9 59.32,15.9 SJ11.1 v59.33,14.65 | SJ11.3 58.32,17.51 58.16,17.67 | SJ10.1 58.33,19.16 58.16,19.32
P5TX_A  (via drill 0.3 pad 0.61)
  Top 0.2: U1.13 55.56,65.34 55.8,65.09 55.8,48.05 v55.55,47.8 | U21.7 68.71,40.73 67.1,42.34 59.61,42.34 v59.36,42.59 59.19,42.76 U22.14
  Top 0.254: U21.7 68.71,35.69 64.18,31.16 64.18,24.3 65.45,23.03 65.45,20.87 64.55,19.97 v60.28,19.97
  Bottom 0.2: v59.36,42.59 56.31,45.64
  Bottom 0.203: 56.31,45.64 55.55,46.4 v55.55,47.8
  Bottom 0.254: SJ10.2 v60.28,19.97
P5TX_B_1.8  (via drill 0.3 pad 0.61)
  Top 0.254: U22.7 59.19,25.66 v58.82,25.29
  Bottom 0.254: SJ9.2 58.19,23.24 57.91,23.52 57.91,24.38 v58.82,25.29
P5TX_B_5  (via drill 0.3 pad 0.61)
  Top 0.254: U21.14 68.71,43.9 70.35,42.26 71.54,42.26 73.05,40.75 73.05,38.49 71.18,36.62 71.18,33.97 68.37,31.16 68.37,25.21 67.23,24.07 67.23,18.46 65.46,16.7 v60.24,16.7
  Bottom 0.254: v60.24,16.7 60.2,16.74 SJ11.2
PHOTORESIST  (via drill 0.3 pad 0.61)
  Top 0.2: U1.90 21.6,68.34 20.14,66.88 20.14,62.18 19.22,61.26 19.22,52.35 v18.69,51.81
  Top 0.406: R16.2 5.84,28.61 R17.1
  Bottom 0.2: R16.2 5.84,41.58 16.07,51.81 v18.69,51.81
PORT1.1  (via drill 0.3 pad 0.61)
  Top 0.2: U1.76 23.9,75.34 23.9,75.33 23.41,74.85 20.7,74.85 20.04,74.19 v20.04,71.48
  Top 0.203: SV1.1 8.23,58.02 v8.23,60.58
  Bottom 0.203: v8.23,60.58 8.23,60.66 19.05,71.48 v20.04,71.48
PORT1.2  (via drill 0.3 pad 0.61)
  Top 0.254: U1.23 45.04,70.34 44.29,69.59 44.29,63.6 41.65,60.96 35.05,60.96 v34.6,60.51
  Bottom 0.254: SV1.2 5.77,55.28 8.55,55.28 10.22,56.94 19.45,56.94 20.62,55.77 28.08,55.77 32.05,59.74 33.83,59.74 v34.6,60.51
PORT1.3  (via drill 0.3 pad 0.61)
  Top 0.254: U1.24 44.6,70.84 44.6,70.81 43.58,69.79 43.58,64 41.19,61.62 v34.53,61.62
  Bottom 0.254: v34.53,61.62 31.38,61.62 26.75,56.99 20.93,56.99 19.93,57.98 8.86,57.98 7.62,59.23 SV1.3
PORT1.4  (via drill 0.3 pad 0.61)
  Top 0.254: U1.9 45.05,63.34 42.06,60.35 35.86,60.35 35.15,59.63 34.03,59.63 33.4,60.27 v33.4,60.76
  Bottom 0.254: SV1.4 5.61,57.98 7.77,57.98 8.3,57.45 19.76,57.45 20.82,56.38 27.24,56.38 31.62,60.76 v33.4,60.76
PORT1.5  (via drill 0.3 pad 0.61)
  Top 0.254: U1.70 29.86,77.93 v29.49,77.56
  Bottom 0.203: SV1.5 22.02,76.88 28.8,76.88 v29.49,77.56
POW1
  Top 0.305: U9.1 U9.2 U9.3
  Top 0.406: U29.3 118.24,50.76 118.28,50.72 118.33,50.76 U29.4
  Top 1.016: U9.2 126.87,20.85 126.84,20.88
  Top 1.422: 129.74,42.58 129.74,39.42 128.01,37.69 125.98,37.69 123.74,35.45 123.74,23.48 122.64,22.38
  Top 1.5: 129.74,42.58 127.47,44.85 121.86,44.85 118.28,48.43 118.28,50.72 118.28,50.85
  Top 1.676: 126.84,20.88 124.14,20.88 122.64,22.38 122.53,22.27 K1.P
POW2
  Top 0.254: 104.43,20.45 104.44,20.45 U6.3
  Top 0.406: 110.66,50.85 110.58,50.76 U30.3 | U30.4 111.3,50.72 110.66,50.72
  Top 0.61: 103.14,22.17 103.24,22.27
  Top 1.27: U6.1 U6.2 104.43,20.59 104.43,20.45
  Top 1.676: 104.44,23.08 U6.1 | K2.P 103.24,22.27 103.63,22.27 104.44,23.08 | 104.44,23.08 110.14,23.08 111.93,24.87 111.93,43.19 110.66,44.46 110.66,50.72 110.66,50.85
POW3
  Top 0.406: U7.3 81.5,20.11 81.58,20.11 81.33,20.37 U7.2 | U32.3 103,50.76 103.04,50.72 103.09,50.76 U32.4
  Top 0.61: U7.2 U7.1 | U7.2 | U7.2 80.79,20.59 | 80.69,21.43 80.87,21.25 81.2,21.25
  Top 1.676: 103.04,50.72 103.04,49.45 92.29,38.69 92.29,30.44 84.88,23.03 82.29,23.03 80.69,21.43 80.69,20.59 | K3.P 73.83,22.27 75.51,20.59 80.69,20.59 | 80.69,20.59 80.79,20.59
POW4
  Top 0.406: U3.3 U3.2 | 49.83,44.75 49.45,44.75 U33.3 | U33.4 49.86,44.46 49.83,44.5
  Top 1.27: 49.83,44.75 49.83,44.5 49.83,42.92 51.1,41.65 51.1,32.1 42.71,23.71 42.71,22.27
  Top 1.5: K4.P 42.71,22.27 U3.1 U3.2
POW5
  Top 0.406: U8.3 25.07,20.08 | 25.07,20.08 25.24,20.08 25.24,21.32 U8.1 | 25.07,20.08 25.07,20.66 U8.2 | 29.38,44.62 29.22,44.46 U34.3 | U34.4 30.01,44.5 29.38,44.5
  Top 1.016: 24.46,20.66 U8.2
  Top 1.5: 29.38,44.62 29.38,44.5 29.38,33.65 21.45,25.72 21.45,22.27
  Top 1.676: 24.46,20.66 24.43,20.67 23.04,20.68 21.45,22.27 K5.P
POW_RAW  (via drill 0.3 pad 0.61)
  Top 0.406: v31.9,33.88 31.9,41.14 36.14,45.39 R77.2
  Top 1.27: 137.54,38.78 R51.1 | 146.1,29.13 146.1,29.49 J10.P$1
  Top 3.8: X2.1 137.26,33.88 138.22,34.84
  Top 3.81: 137.54,38.78 PC5.+ 138.86,38.78 138.22,38.15 138.22,34.84 138.22,31.16 140.25,29.13 146.1,29.13
  Bottom 3.81: X2.1 X3.1 X4.1 X5.1 v31.9,33.88 X6.1
RESET_OUTPUT  (via drill 0.3 pad 0.61)
  Top 0.254: v71.12,80.67 66.85,80.67 66.13,81.39 66.13,81.72 U25.8
  Top 0.3: R11.1 124.01,80.81 123.62,81.2 116.73,81.2
  Top 0.305: 116.73,81.2 114.88,79.34 v105.25,79.34
  Top 0.406: 66.13,81.72 R58.2
  Bottom 0.254: v71.12,80.67 99.56,80.67 101.39,82.49 102.81,82.49 105.25,80.06 v105.25,79.34
RESET_OUTPUT_ERASE
  Bottom 0.254: U37.8 90.4,95.85 R104.2 89.44,98.65 106.67,98.65 109.01,96.32 135.42,96.32 136.95,94.79 136.95,87.17 137.66,86.46 141.22,86.46 141.53,86.15 U38.1
RESET_OUTPUT_PCMR
  Bottom 0.254: U40.8 101.59,95.04 | 101.59,95.04 99.41,95.04 98.89,95.56 R111.2 | SJ15.2 101.49,95.14 101.59,95.04
  Bottom 0.508: SJ16.2 103.98,95.8 U40.8
RESET_OUTPUT_PCMR_POW
  Bottom 0.254: SJ15.1 100.68,98.04 100.78,98.14 102.2,98.14 102.31,98.04 SJ15.3 102.2,97.12 102.51,97.43 106.99,97.43 108.61,95.81 134.81,95.81 136.14,94.48 136.14,92.65 133.09,89.6 133.09,87.37 133.6,86.86 135.43,86.86 135.83,86.46 135.83,81.48 136.85,80.46 139.19,80.46 140.72,78.94 R113.1
RESET_OUTPUT_PCMR_RST
  Bottom 0.254: U39.1 133.29,85.64 132.48,86.46 132.48,90.11 135.63,93.26 135.63,94.18 134.51,95.3 106.78,95.3 | SJ16.3 106.47,94.99 106.78,95.3 | SJ16.1 106.57,96.62 106.78,96.41 106.78,95.3
RXL  (via drill 0.3 pad 0.61)
  Top 0.2: 40.22,50.59 v40.37,50.74 39.81,50.19 32.61,50.19 30.58,52.22 30.58,54.76 30.27,55.06 28.05,55.06 27.24,55.88 27.24,58.38 30.07,61.21 30.07,61.77 29.56,62.28 28.34,62.28 27.9,61.84 U1.103 | RX.C 136.99,97.53 135.5,97.53 135.22,97.26 135.22,94.18 v134.41,93.37
  Top 0.254: v131.97,85.64 128.21,81.88 v127.3,81.88
  Bottom 0.254: v40.37,50.74 40.91,51.28 49.88,51.28 51.48,52.88 89.24,52.88 94.27,57.91 102.51,57.91 112.16,67.56 112.16,75.8 118.07,81.71 127.12,81.71 v127.3,81.88 | v134.41,93.37 131.97,90.93 v131.97,85.64
SCL_3  (via drill 0.3 pad 0.61)
  Top 0.2: U4.6 16.94,68.28 17.14,68.08 18.84,68.08 20.6,69.84 U1.87 27.77,69.84 29.36,68.25 v30.53,68.25
  Top 0.254: U2.6 97.56,82.19 97.18,81.82 97.18,75.81 v97.71,75.28 v114.73,75.28 | U15.8 131.86,64.18 v131.86,63.43 v131.85,63.42 | U11.6 141.74,84.38 140.64,83.28 136.64,83.28 135.44,82.08 v135.44,73.88 | U4.6 | U17.8 120.53,64.35 v120.57,64.31 124.26,64.31 v124.39,64.18
  Top 0.406: U4.6 R1.1
  Bottom 0.2: v97.71,75.28 96.79,75.28 95.47,73.96 63.67,73.96 60.42,70.71 44.19,70.71 42.87,72.03 37.36,72.03 33.57,68.25 v30.53,68.25
  Bottom 0.254: v135.44,73.88 136.74,73.88 137.34,73.28 137.34,66.18 134.58,63.42 v131.85,63.42 125.15,63.42 v124.39,64.18 | v120.57,64.31 120.57,69.44 v114.73,75.28
SD_CD  (via drill 0.3 pad 0.61)
  Top 0.254: U1.72 28.86,82.91 v29.13,83.18 | v88.16,83.61 91.38,83.61 X7.CD1 | v52.56,90.11 v47.44,90.11
  Bottom 0.254: v52.56,90.11 60.25,90.11 62.28,88.08 73.66,88.08 77.92,83.81 87.95,83.81 v88.16,83.61 | v47.44,90.11 36.06,90.11 35.47,89.52 31.5,89.52 30.58,88.6 30.58,84.63 29.56,83.61 v29.13,83.18
SD_CS  (via drill 0.3 pad 0.61)
  Top 0.254: U1.71 29.36,81.6 v29.64,81.88 | v73.44,87.08 76.2,89.83 IC1.7 | v52.65,89.01 v47.44,89.01
  Bottom 0.254: v73.44,87.08 62.36,87.08 60.45,89 53.89,89 v52.65,89.01 | 29.97,82.21 v29.64,81.88 31.09,83.32 31.09,88.39 31.71,89.01 v47.44,89.01
SD_DI  (via drill 0.3 pad 0.61)
  Top 0.2: U1.109 28.86,58.07 32.81,62.02 v32.81,62.66 | IC1.5 75.2,87.3 74.37,86.46 74.37,83.41 72.44,81.48 v67.46,81.48
  Bottom 0.2: v32.81,62.66 32.43,62.28 28.75,62.28 28.14,62.89 28.14,69.19 32.81,73.86 44.34,73.86 45.87,72.33 54.76,72.33 63.9,81.48 v67.46,81.48
SD_DO  (via drill 0.3 pad 0.61)
  Top 0.2: U1.108 27.54,59.34 29.05,60.85 v29.05,61.46
  Top 0.254: X7.7 90.99,95.41 89.78,96.62 84.12,96.62 79.45,91.94 75.59,91.94 v73.25,89.61 | v63.9,89 v63.9,83.31
  Bottom 0.2: v63.9,83.31 63.9,82.34 54.3,72.74 46.35,72.74 44.83,74.27 32.51,74.27 27.53,69.29 27.53,62.68 28.75,61.46 v29.05,61.46
  Bottom 0.305: v63.9,89 72.64,89 v73.25,89.61
SD_SCK  (via drill 0.3 pad 0.61)
  Top 0.2: U1.110 29.36,57.97 33.7,62.31 33.7,63.42 32.81,64.31 v32.81,67.36 | IC1.3 76.42,84.75 71.42,79.75 v69.69,79.75 v64.11,79.75 | v69.09,83.51 69.08,83.81 69.08,87.37 68.58,87.88 68.58,90.01 69.67,91.1 IC1.9
  Bottom 0.2: v32.81,67.36 29.64,67.36 29.05,67.94 29.05,69.39 33.12,73.45 43.86,73.45 45.39,71.93 55.16,71.93 62.99,79.75 v64.11,79.75
  Bottom 0.254: v69.69,79.75 69.29,80.16 69.29,83.31 v69.09,83.51
SDA_3  (via drill 0.3 pad 0.61)
  Top 0.2: R12.1 18.92,71.08 19.04,71.08 19.78,70.34 U1.86 28.69,70.34 v29.89,69.13
  Top 0.254: U2.5 96.29,82.52 96.58,82.22 96.58,74.86 v97.21,74.23 v113.71,74.23 | U17.7 v115.65,64.35 116.61,63.38 126.81,63.38 127.17,63.74 U15.7 129.15,64.22 v129.21,64.28 | U11.1 141.54,81.58 140.64,82.48 137.24,82.48 136.54,81.78 136.54,73.38 v136.14,72.98
  Top 0.406: U4.5 18.21,71.03 R12.1
  Bottom 0.2: v97.21,74.23 97.98,74.23 98.6,74.85 98.6,75.61 98.09,76.12 96.77,76.12 95.06,74.41 63.23,74.41 59.94,71.11 44.6,71.11 43.17,72.54 36.98,72.54 33.57,69.13 v29.89,69.13
  Bottom 0.254: 136.14,73.03 v136.14,72.98 136.14,66.28 134.14,64.28 v129.21,64.28 | v115.65,64.35 118.28,66.98 118.28,69.66 v113.71,74.23
THM0  (via drill 0.3 pad 0.61)
  Top 0.254: U17.3 109.41,69.43 108.99,69.01 108.99,62.77 108,61.77 99.87,61.77 98.98,60.88 v98.98,55.55 | JP2.2 64.69,9.96 R87.2 66.24,10.59 v66.72,10.59 | v88.79,43.68 88.79,42.97 88.18,42.36 88.18,35.05 80.41,27.27 80.41,23.81 79.35,22.55 76.6,22.55 v76.25,22.91
  Bottom 0.254: v98.98,55.55 98.98,50.47 96.31,47.8 91.11,47.8 88.79,45.49 v88.79,43.68 | v76.25,22.91 66.72,13.38 v66.72,10.59
TXL  (via drill 0.3 pad 0.61)
  Top 0.203: TX.C 135.82,98.63 134.72,97.53 133.29,97.53 132.99,97.23 132.99,84.83 129.23,81.07 v127.55,81.07
  Top 0.254: U1.107 25.9,59.84 25.64,59.58 25.64,57.66 26.21,57.09 26.21,55.27 29.76,51.71 30.27,51.71 32.3,49.68 v40.81,49.68 v40.8,49.67 | TX.C 136.19,98.6 135.99,98.6
  Bottom 0.254: v127.55,81.07 118.77,81.07 112.77,75.08 112.77,67.36 102.71,57.3 94.96,57.3 90.03,52.37 51.86,52.37 50.27,50.78 41.91,50.78 v40.8,49.67
VBAT
  Top 0.61: C13.1 97.99,87.31 97.56,87.74 U2.3
  Top 0.813: C13.1 R21.1
VBG
  Top 0.2: C25.1 51.95,81.38 46.53,81.38 44.86,79.71 U1.40
  Top 0.254: C25.1 R8.1
VDDANA
  Top 0.254: U1.73 26.28,76.84 25.8,77.31 25.8,79.27 L1.2
  Top 0.406: L1.2 25.5,79.63 C26.1 25.46,80.79 C36.+
VDDOUT  (via drill 0.3 pad 0.61)
  Top 0.2: U1.45
  Top 0.254: C27.1 C32.1 35.49,54.69 | U1.104 24.87,61.34 C33.1 | U1.56 36.86,79.96 v36.84,79.98 36.76,80.06 36.57,80.06 35.04,81.59 C28.1 35.04,81.47 34.36,80.79 34.36,80.16 | 35.49,54.69 36.36,55.56 U1.124 36.36,58.91 37.18,59.74 42.46,59.74 v45.21,62.48 | v45.31,64.31 45.78,63.84 U1.10 49.13,63.84 50.22,62.75 C34.1 | U1.45 42.36,77.82 42.16,77.62 40.74,77.62 40.43,77.31 40.43,75.48 43.17,72.74 43.17,70.71 42.57,70.1 v42.57,64.41 | 35.49,54.69 35.49,55.43 34.95,55.98 32.51,55.98 v32.3,55.77 | v29.15,54.25 28.14,54.25 26.72,55.67 26.72,57.7 v26.41,58.01 | U1.45 42.36,79.75 42.67,80.06 v42.67,81.09 42.67,81.77 C35.1 42.77,81.87 | L5.1 33.06,79.98 34.18,79.98 34.36,80.16 | U1.61 34.36,80.16
  Top 0.3: C33.1 23.6,61.6 v23.57,61.57
  Top 0.406: C8.+ 22.62,62.51 v23.57,61.57
  Bottom 0.254: v45.21,62.48 45.21,64.21 v45.31,64.31 45.21,64.41 v42.57,64.41 | v32.3,55.77 30.78,54.25 v29.15,54.25 | v42.67,81.09 41.43,79.85 36.97,79.85 v36.84,79.98
  Bottom 0.3: v26.41,58.01 26.41,58.72 v23.57,61.57
VDDOUTMI
  Top 0.254: C37.+ 46.75,82.37 45.72,82.37 45.72,81.27 44.36,79.92 U1.41
  Top 0.61: C37.+ 47.36,82.98 C20.1
  Top 0.8: 45.72,82.37 L2.2
VDDPLL  (via drill 0.3 pad 0.61)
  Top 0.254: C39.+ 52.16,74.77 51.61,74.77 50.55,75.84 U1.34 43.23,75.84 v42.36,76.7 | L5.2 31.85,83.57 32.61,84.32 36.06,84.32 v36.17,84.22
  Top 0.406: C39.+ 54.5,74.09 C38.1
  Bottom 0.254: v42.36,76.7 42.36,78.73 41.85,79.24 36.27,79.24 35.96,79.55 35.96,84.02 v36.17,84.22
VIN_5
  Top 0.61: U28.1 U28.2 124.31,50.69 123.74,50.69
  Top 1.5: R51.2 134.21,41.65 128.42,47.44 124.56,47.44 123.74,48.26 123.74,50.69
VIN_BRD  (via drill 0.3 pad 0.61)
  Top 0.152: v128.78,51.82 128.78,52.42 | 128.78,52.42 v128.68,52.52 128.78,52.42 | v129.48,52.42 128.78,52.42
  Top 0.406: K3.2 75.99,28.24 78.33,30.58 78.33,42.46 80.17,44.3 U10.10
  Top 0.61: 126.18,50.76 U28.3
  Top 1.016: U5.3 138.4,51.54 138.44,51.58
  Top 1.27: U28.4 126.19,50.76 126.18,50.76
  Top 1.676: 138.44,51.58 138.44,54.03 F1.2
  Top 1.778: U28.4 v128.68,52.52 130.19,54.03 PC2.+
  Top 1.93: PC2.+ 138.34,54.03 F1.2
  Bottom 1.5: K1.2 119.17,29.76 118.41,30.53 | 118.41,30.53 97.2,30.53 | 97.2,30.53 74.09,30.53 | 74.09,30.53 41.07,30.53 | 41.07,30.53 23.03,30.53 20.75,28.24 K5.2 | K4.2 40.05,29.51 41.07,30.53 | K3.2 73.2,29.64 74.09,30.53 | K2.2 96.19,29.51 97.2,30.53 | 118.41,30.53 133.75,30.53 135.68,32.46 135.68,45.51 v128.68,52.52
VUSBD
  Top 0.406: J3.1 8.33,51.51 9.16,52.34 C30.+
  Top 1.27: C30.+ 9.16,56.06 F2.1
XIN
  Top 0.254: U1.36 50.72,76.84 52.55,78.67 Y1.1 52.78,79.7 53.13,80.06 55.47,80.06 55.88,79.64 C22.1
XIN32
  Top 0.254: U1.48 40.86,84.95 42.16,86.25 Y2.P$2 | Y2.P$2 42.16,88.73 C24.1 | Y2.P$2
XOUT
  Top 0.2: Y1.3 C21.2
  Top 0.254: U1.35 50.92,76.34 52.12,77.54 53.72,77.54 54.32,76.94 54.32,76.77 Y1.3
XOUT32
  Top 0.254: U1.49 40.36,84.97 39.06,86.27 Y2.P$1 39.06,88.73 C23.1
XU4_MEDIA_SEL_IN  (via drill 0.3 pad 0.61)
  Top 0.406: v17.77,42.26 19.3,42.26 21.23,44.19 21.23,44.52 R32.1
  Bottom 0.406: U14.1 11.42,36.53 10.97,36.98 10.97,40.43 11.48,40.94 12.89,40.94 U13.1 16.46,40.95 v17.77,42.26
XUSB  (via drill 0.3 pad 0.61)
  Top 0.3: v45.13,77.39 45.36,77.62 U1.39
  Top 0.406: F2.2 11.35,61.94 12.26,61.03 v12.26,60.93
  Bottom 0.406: v45.13,77.39 45.13,77.26 43.61,75.74 23.72,75.74 22.27,74.29 22.27,71.62 13.81,63.16 13.78,63.16 12.26,61.65 v12.26,60.93

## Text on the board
tNames: http://wa8.gl/system/wagman/wagman-v4.0.html | - | + | Wagman V4.0 | 09/2018
DrillLegend: LAYER-STACK
DrillLegend_01-16: 01-16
